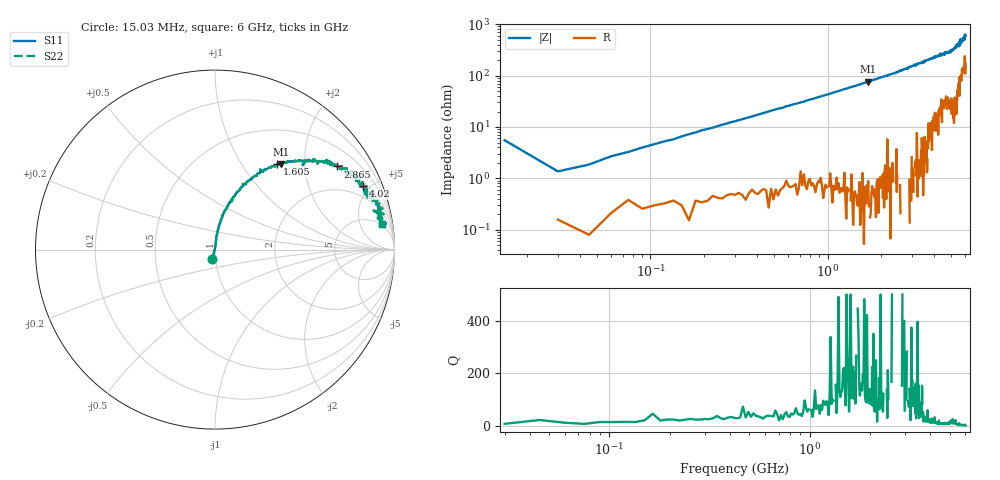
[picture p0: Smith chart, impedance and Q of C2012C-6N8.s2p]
!	Network	Analyzer	HP8753E.07.74:	Oct	30	2002	Serial	No.	JP38451487
!	Hewlett-Packard
!	7	Sep	2009	10:41:17
!	Frequency	S11	S21	S12	S22
#	HZ	S	RI	R	50
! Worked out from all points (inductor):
!   400 points, 15.03 MHz to 6 GHz, reference 50 ohm
!   read as one part in series: L = 6.91 nH near 45.03 MHz
!   highest Q = 205 at 1.695 GHz (marker M1), where L = 7.17 nH
!   S11 on the Smith chart (normalised r, x): 15.03 MHz: 0.96, -0.10; 1.605 GHz: 1.00, +1.45; 2.865 GHz: 1.02, +2.94; 4.02 GHz: 1.23, +4.53; 6 GHz: 4, +11
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1.502992e7  -0.0151 -0.0536  1.02 0.0536  1.02 0.0536  -0.0151 -0.0536
3.002985e7  0.00154 0.0136  0.998 -0.0136  0.998 -0.0136  0.00154 0.0136
6.00297e7  0.00268 0.0268  0.997 -0.0268  0.997 -0.0268  0.00268 0.0268
1.200294e8  0.00599 0.0521  0.994 -0.0521  0.994 -0.0521  0.00599 0.0521
2.850286e8  0.0198 0.121  0.98 -0.121  0.98 -0.121  0.0198 0.121
5.850271e8  0.0685 0.235  0.932 -0.235  0.932 -0.235  0.0685 0.235
1.020025e9  0.166 0.364  0.834 -0.364  0.834 -0.364  0.166 0.364
1.605022e9  0.345 0.475  0.655 -0.475  0.655 -0.475  0.345 0.475
1.695022e9  0.37 0.477  0.63 -0.477  0.63 -0.477  0.37 0.477
2.01002e9  0.462 0.494  0.538 -0.494  0.538 -0.494  0.462 0.494
2.865016e9  0.682 0.463  0.318 -0.463  0.318 -0.463  0.682 0.463
3.015015e9  0.707 0.466  0.293 -0.466  0.293 -0.466  0.707 0.466
4.00501e9  0.835 0.353  0.165 -0.353  0.165 -0.353  0.835 0.353
4.02001e9  0.825 0.355  0.175 -0.355  0.175 -0.355  0.825 0.355
5.010005e9  0.884 0.282  0.116 -0.282  0.116 -0.282  0.884 0.282
5.445003e9  0.922 0.214  0.0776 -0.214  0.0776 -0.214  0.922 0.214
5.535002e9  0.884 0.217  0.116 -0.217  0.116 -0.217  0.884 0.217
5.565002e9  0.94 0.198  0.0602 -0.198  0.0602 -0.198  0.94 0.198
5.595002e9  0.899 0.209  0.101 -0.209  0.101 -0.209  0.899 0.209
5.625002e9  0.932 0.173  0.0681 -0.173  0.0681 -0.173  0.932 0.173
5.715001e9  0.912 0.191  0.0878 -0.191  0.0878 -0.191  0.912 0.191
6e9  0.93 0.144  0.0698 -0.144  0.0698 -0.144  0.93 0.144
